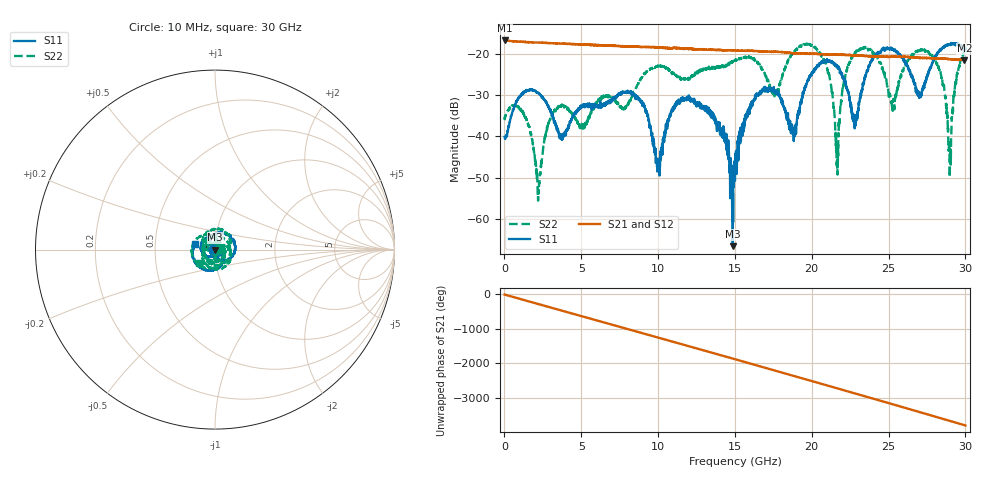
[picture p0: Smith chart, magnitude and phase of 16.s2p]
#  HZ  S  DB  R  50.00
! Rohde & Schwarz Vector Network Analyzer
! Rohde-Schwarz,ZNB40-4Port,1311601084101679,3.45
! Created: UTC 10/20/2022, 5:24:35 PM
! freq[Hz]  db:S11  ang:S11  db:S31  ang:S31  db:S13  ang:S13  db:S33  ang:S33
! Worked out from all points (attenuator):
!   3000 points, 10 MHz to 30 GHz, reference 50 ohm
!   highest |S21| = -16.84 dB at 20 MHz (marker M1); lowest = -21.6 dB at 29.94 GHz (marker M2)
!   lowest |S11| = -66.5 dB at 14.86 GHz (marker M3), VSWR 1.00, Z = 50 + j0.0344 ohm
!   |S11| at or under -10 dB: start of sweep to end of sweep
!   |S22| runs from -55.5 to -17.6 dB; largest |S21 - S12| = 0.0029
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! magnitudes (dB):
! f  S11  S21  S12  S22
! 10 MHz  -40.1  -16.8  -16.8  -35.5
! 20 MHz  -40.3  -16.8  -16.8  -35.8
! 1.3 GHz  -29.3  -17.2  -17.2  -34.7
! 2.21 GHz  -29.4  -17.4  -17.4  -54.0
! 3.28 GHz  -36.5  -17.5  -17.5  -33.5
! 5.01 GHz  -33.1  -17.8  -17.8  -37.7
! 8.36 GHz  -29.5  -18.3  -18.4  -29.9
! 10.01 GHz  -46.0  -18.5  -18.6  -23.0
! 12.02 GHz  -30.4  -18.8  -18.9  -26.3
! 14.86 GHz  -66.5  -19.2  -19.2  -21.8
! 15.01 GHz  -48.2  -19.2  -19.2  -21.7
! 16.44 GHz  -30.1  -19.4  -19.4  -22.0
! 17.59 GHz  -29.3  -19.6  -19.6  -29.8
! 18.84 GHz  -39.2  -19.9  -19.9  -19.7
! 20.01 GHz  -24.7  -20.1  -20.1  -18.0
! 21.64 GHz  -22.8  -20.2  -20.2  -45.3
! 22.91 GHz  -34.8  -20.5  -20.4  -19.4
! 25.01 GHz  -18.9  -20.8  -20.8  -30.2
! 27.69 GHz  -23.4  -21.1  -21.1  -20.2
! 28.98 GHz  -17.8  -21.4  -21.3  -49.9
! 29.94 GHz  -18.7  -21.6  -21.6  -19.2
! 30 GHz  -18.8  -21.5  -21.6  -18.6
